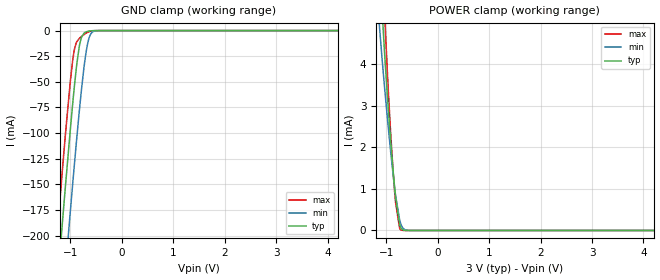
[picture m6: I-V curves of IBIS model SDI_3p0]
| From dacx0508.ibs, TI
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|   Model
[Model]   SDI_3p0
Model_type   Input
Vinl = 0.9
Vinh = 2.1
|   typ   min   max
C_comp   1.15784pF   1.04626pF   1.19578pF
| Where nom  PVT is Nominal Process, 3.0V, 27C
|   Fast PVT is Strong Process,  3.3V, -40C
|   Slow PVT is Weak Process,   2.7V, 125C
[Voltage Range]   3   2.7   3.3
|Junction Temperature
[Temperature Range]   27   125   -40
[Power Clamp Reference]   3   2.7   3.3
[GND Clamp Reference]   0   0   0
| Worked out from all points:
|   GND clamp passes 1 mA (typ) near -0.68 V on its own axis
|   POWER clamp passes 1 mA (typ) near -0.84 V on its own axis
[GND Clamp]
|   Voltage   I(typ)   I(min)   I(max)
-3V       -1.382A    -1.46A     -1.333A
-1.326V   -292.7mA   -375mA     -240.8mA
-1.164V   -192.1mA   -274.2mA   -140.6mA
-1.101V   -154mA     -235.6mA   -103.3mA
-1.002V   -96.43mA   -176.3mA   -49.33mA
-930mV    -57.79mA   -134.5mA   -20.39mA
-876mV    -32.61mA   -104.4mA   -10.87mA
-813mV    -11.72mA   -71.17mA   -6.994mA
-696mV    -1.312mA   -21.17mA   -2.523mA
-615mV    -301.4uA   -4.293mA   -708.7uA
-480mV    -11.64uA   -115.4uA   -19.78uA
6V        0A         0A         0A
[POWER Clamp]
|   Voltage   I(typ)   I(min)   I(max)
-3V       56.91mA    44.69mA    68.98mA
-1.146V   6.755mA    5.097mA    8.527mA
-1.083V   5.308mA    4.135mA    6.651mA
-1.047V   4.539mA    3.62mA     5.617mA
-1.02V    3.995mA    3.247mA    4.869mA
-921mV    2.245mA    1.962mA    2.454mA
-840mV    1.051mA    1.041mA    956.8uA
-822mV    825.1uA    862.5uA    691.1uA
-741mV    143.2uA    256uA      49.82uA
-705mV    43.88uA    117uA      9.199uA
-516mV    17.29nA    598.5nA    0A
6V        0A         0A         0A
